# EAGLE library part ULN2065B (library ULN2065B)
ULN2065B, Darlington Transistor Array, NPN 1.75 A 80 V, Quad, 16-Pin, Power PDIP Source: Datasheet
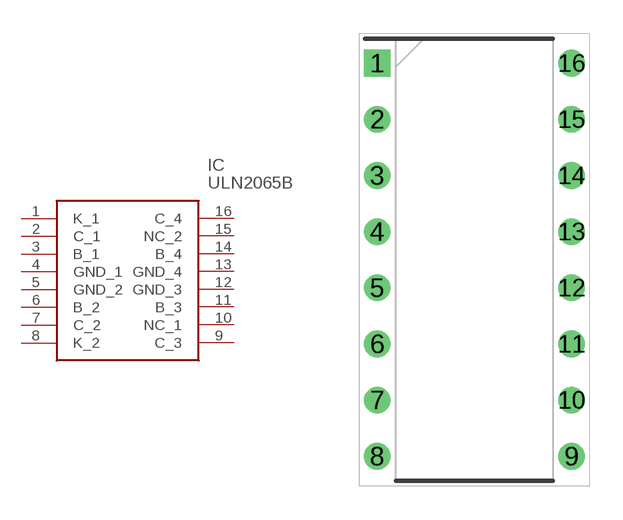
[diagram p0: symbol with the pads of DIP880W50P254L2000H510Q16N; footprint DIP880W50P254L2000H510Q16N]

Designator prefix IC

## ULN2065B (Arrow_Part_Number: ULN2065B; Arrow_Price-Stock: https://www.arrow.com/en/products/uln2065b/stmicroelectronics?utm_currency=USD&region=europe; Description: ULN2065B, Darlington Transistor Array, NPN 1.75 A 80 V, Quad, 16-Pin, Power PDIP; Height: 5.1mm; Manufacturer_Name: STMicroelectronics; Manufacturer_Part_Number: ULN2065B; Mouser_Part_Number: 511-ULN2065B; Mouser_Price-Stock: https://www.mouser.co.uk/ProductDetail/STMicroelectronics/ULN2065B?qs=FOlmdCx%252BAA2jqcA5kVo46g%3D%3D)  [DIP880W50P254L2000H510Q16N]
1  K_1
2  C_1
3  B_1
4  GND_1
5  GND_2
6  B_2
7  C_2
8  K_2
9  C_3
10  NC_1
11  B_3
12  GND_3
13  GND_4
14  B_4
15  NC_2
16  C_4

## Footprint DIP880W50P254L2000H510Q16N (pad centres in mm)
Power DIP16
drill 0.7 pad 1.1 square: 1 -4.4,8.89
drill 0.7 pad 1.1: 2 -4.4,6.35; 3 -4.4,3.81; 4 -4.4,1.27; 5 -4.4,-1.27; 6 -4.4,-3.81; 7 -4.4,-6.35; 8 -4.4,-8.89; 9 4.4,-8.89; 10 4.4,-6.35; 11 4.4,-3.81; 12 4.4,-1.27; 13 4.4,1.27; 14 4.4,3.81; 15 4.4,6.35; 16 4.4,8.89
